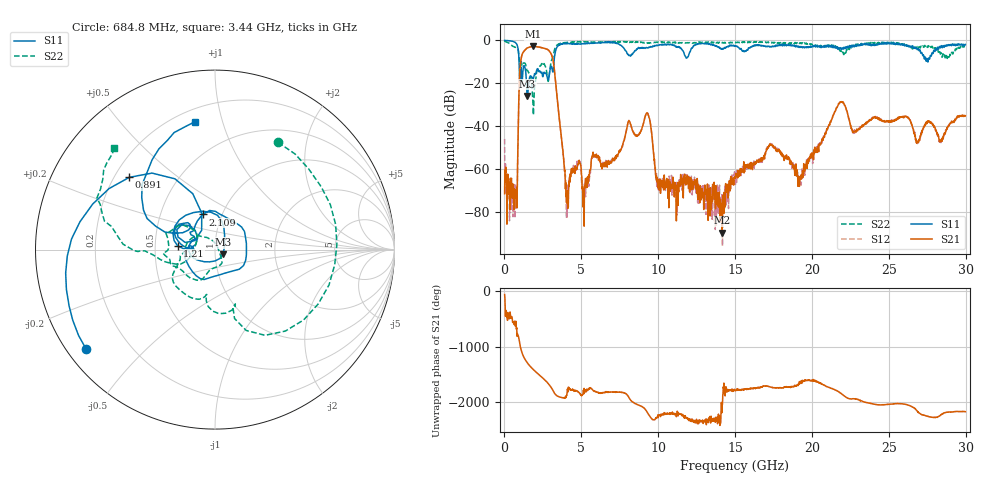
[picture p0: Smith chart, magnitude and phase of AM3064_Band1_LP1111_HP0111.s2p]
# Hz S DB R 50.0
!freq dBS11 angS11 dBS21 angS21 dBS12 angS12 dBS22 angS22
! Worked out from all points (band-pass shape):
!   1600 points, 10 MHz to 29.98 GHz, reference 50 ohm
!   highest |S21| = -2.81 dB at 1.884 GHz (marker M1); lowest = -89.6 dB at 14.16 GHz (marker M2)
!   |S21| within 3 dB of the highest: 1.193 GHz to 2.998 GHz (1.804 GHz wide, 86.1 % of centre)
!   lowest |S11| = -25.9 dB at 1.491 GHz (marker M3), VSWR 1.11, Z = 54.4 - j2.95 ohm
!   |S11| at or under -10 dB: 949.7 MHz to 3.222 GHz (2.272 GHz wide, 109 % of centre); 27.5352 GHz to 27.54622 GHz (11.02 MHz wide, 0.04 % of centre)
!   |S22| runs from -34.8 to -0.2 dB; largest |S21 - S12| = 0.011
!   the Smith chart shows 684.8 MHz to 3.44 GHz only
!   S11 on the Smith chart (normalised r, x): 684.8 MHz: 0.05, -0.34; 891 MHz: 0.26, +0.34; 1.21 GHz: 0.66, +0.03; 2.109 GHz: 0.81, +0.33; 3.44 GHz: 0.28, +0.82
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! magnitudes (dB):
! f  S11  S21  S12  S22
! 10 MHz  0.0  -71.4  -45.9  -0.2
! 684.8 MHz  -0.8  -71.5  -82.8  -3.2
! 891 MHz  -4.1  -42.9  -43.0  -4.4
! 1.041 GHz  -13.2  -10.7  -10.6  -8.9
! 1.21 GHz  -13.6  -5.6  -5.6  -11.1
! 1.491 GHz  -25.9  -3.5  -3.4  -14.1
! 1.884 GHz  -17.7  -2.8  -2.9  -34.8
! 2.109 GHz  -13.7  -3.0  -3.0  -14.3
! 3.028 GHz  -12.1  -6.2  -6.2  -10.2
! 3.44 GHz  -2.8  -27.6  -27.5  -2.0
! 4.059 GHz  -1.4  -72.8  -67.0  -0.9
! 5.015 GHz  -1.6  -62.8  -66.2  -0.5
! 9.269 GHz  -3.4  -33.7  -33.6  -1.3
! 10 GHz  -2.2  -67.8  -69.9  -0.9
! 14.16 GHz  -3.9  -89.6  -85.1  -0.9
! 15 GHz  -2.6  -63.4  -65.5  -1.2
! 19.99 GHz  -3.2  -53.1  -52.8  -1.6
! 21.87 GHz  -3.6  -28.7  -28.9  -4.8
! 22.75 GHz  -3.0  -42.6  -42.7  -1.9
! 25 GHz  -1.1  -38.0  -37.5  -1.1
! 28.41 GHz  -2.4  -46.6  -46.1  -5.8
! 29.98 GHz  -1.9  -35.1  -35.0  -2.9
